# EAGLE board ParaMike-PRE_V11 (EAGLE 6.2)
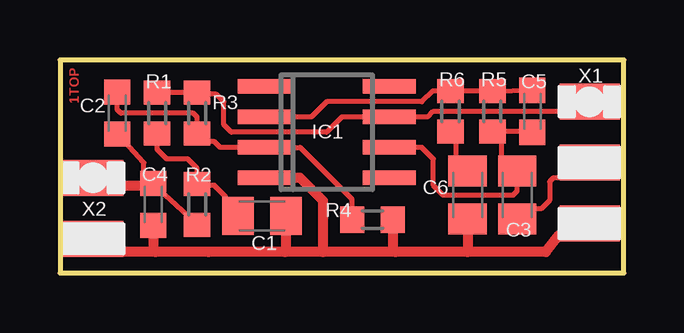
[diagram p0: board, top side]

Size 23.5 x 8.89 mm. Coordinates in mm from the lower left corner, seen from the top.
Outline: 0,8.89 0,0 23.5,0 23.5,8.89 0,8.89
Copper layers (1*16): Top 0.035mm / dielectric 1.5mm / Bottom 0.035mm
Design rules: minimum track width 6mil, minimum drill 12mil, track to track 6mil, track to pad 6mil, pad to pad 6mil, via to via 6mil, smd to smd 6mil, copper to edge 20mil, drill to drill 8mil, minimum pad ring 8mil, minimum via ring 6mil, stop-mask expansion 3mil, vias tented up to drill 0mil, thermal gap 8mil

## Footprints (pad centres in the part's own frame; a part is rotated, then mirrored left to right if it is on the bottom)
C0805K = smd 1.3 x 1.6: 1 -1,0; 2 1,0
C0603K = smd 1.05 x 1.08: 1 -0.875,0; 2 0.875,0
SO08 = smd 0.6 x 2.2: 1 -1.905,-2.6; 2 -0.635,-2.6; 3 0.635,-2.6; 4 1.905,-2.6; 5 1.905,2.6; 6 0.635,2.6; 7 -0.635,2.6; 8 -1.905,2.6
R0603 = smd 1 x 1.1: 1 -0.85,0; 2 0.85,0
AKK3PAD-HALF = smd 2.5 x 1.5: 1 0,2.54; 2 0,0; 3 0,-2.54
AKK2PAD-HALF = smd 2.5 x 1.5: 1 0,1.27; 2 0,-1.27

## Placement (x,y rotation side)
C1  1u  [C0805K]  8.41,2.38 180 top
C2  22n  [C0603K]  2.38,6.67 90 top
C3  220n  [C0805K]  19.05,3.25 270 top
C4  100p  [C0603K]  3.89,2.86 270 top
C5  1n  [C0603K]  19.68,6.75 90 top
C6  2u2  [C0805K]  16.99,3.25 270 top
IC1  LT1007CS8  [SO08]  11.11,5.87 270 top
R1  4k7  [R0603]  4.05,6.67 90 top
R2  4k7  [R0603]  5.71,2.86 90 top
R3  47k  [R0603]  5.71,6.67 90 top
R4  47k  [R0603]  13.02,2.22 180 top
R5  22k  [R0603]  18.02,6.75 270 top
R6  220E  [R0603]  16.27,6.75 90 top
X1  AKK3PAD-HALF  [AKK3PAD-HALF]  22.07,4.6 0 top
X2  AKK2PAD-HALF  [AKK2PAD-HALF]  1.38,2.7 0 top

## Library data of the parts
C1 C3 C6 = rcl; SIZE: 0805
C2 C4 C5 R1 R2 R5 = rcl
IC1 = linear
R3 R4 R6 = rcl; TYPE: THIN FILM
X1 X2 = Akki_V6

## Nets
+BAT: IC1.7 R1.2 R3.2 X1.1
GND: C1.1 C4.2 C6.2 IC1.4 R4.1 X1.3 X2.2
N$1: C6.1 R6.1
N$2: C2.2 IC1.3 R3.1 R4.2
N$3: C5.2 IC1.2 R5.1 R6.2
N$4: C3.1 C5.1 IC1.6 R5.2
N$5: C3.2 X1.2
N$6: C2.1 C4.1 R2.1 X2.1
N$7: C1.2 R1.1 R2.2

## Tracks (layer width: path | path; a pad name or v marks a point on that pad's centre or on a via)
+BAT
  Top 0.203: X1.1 21.67,6.75 15.56,6.75 15.32,6.51 IC1.7 11.75,6.51 11.11,5.87 7.14,5.87 6.83,6.19 6.83,7.14 6.51,7.46 5.77,7.46 R3.2 R1.2
GND
  Top 0.406: 16.99,0.87 20.24,0.87 20.8,1.59 21.75,1.59 X1.3 | C6.2 16.99,0.87 | 16.99,0.87 13.97,0.87 | 13.97,0.87 10.95,0.87 | 10.95,0.87 9.37,0.87 | 9.37,0.87 6.19,0.87 | X2.2 2.25,0.87 3.97,0.87 | IC1.4 10,3.97 10.95,3.02 10.95,0.87 | 6.19,0.88 6.19,0.87 | C1.1 9.41,0.92 9.37,0.87 | R4.1 13.87,0.98 13.97,0.87 | 6.19,0.87 3.97,0.87 | C4.2 3.89,0.95 3.97,0.87
N$1
  Top 0.203: C6.1 16.99,4.29 16.51,4.76 16.51,5.66 R6.1
N$2
  Top 0.203: C2.2 2.38,6.83 2.54,6.67 5.56,6.67 5.71,6.51 R3.1 6.06,5.48 6.43,5.48 6.67,5.24 IC1.3 10,5.24 12.17,3.07 R4.2
N$3
  Top 0.203: C5.2 R5.1 R6.2 15.53,7.6 15.08,7.14 11.11,7.14 10.48,6.51 IC1.2
N$4
  Top 0.203: C5.1 19.66,5.9 R5.2 18.41,5.9 18.41,4.76 C3.1 19.05,3.41 18.89,3.25 15.95,3.25 15.56,3.65 15.56,4.76 15.08,5.24 IC1.6
N$5
  Top 0.203: X1.2 21.75,4.6 21.27,3.97 20.56,3.97 20.4,3.81 20.4,3.02 20.08,2.7 19.53,2.7 19.08,2.25 C3.2
N$6
  Top 0.203: R2.1 5.69,2.01 5.32,2.38 4.37,3.25 C4.1 3.49,4.13 3.49,4.6 2.7,5.48 2.7,5.47 C2.1
  Top 0.406: X2.1 1.91,3.97 2.22,3.65 3.81,3.65 C4.1
N$7
  Top 0.203: R1.1 4.05,5.16 4.45,4.76 5.32,4.76 5.71,4.37 R2.2 5.77,3.65 6.43,3.65 6.91,3.17 6.91,3.02 7.41,2.51 C1.2

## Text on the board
Top: 1TOP
tDocu: (c) ASkr | ParaMike V1.1 | PRE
